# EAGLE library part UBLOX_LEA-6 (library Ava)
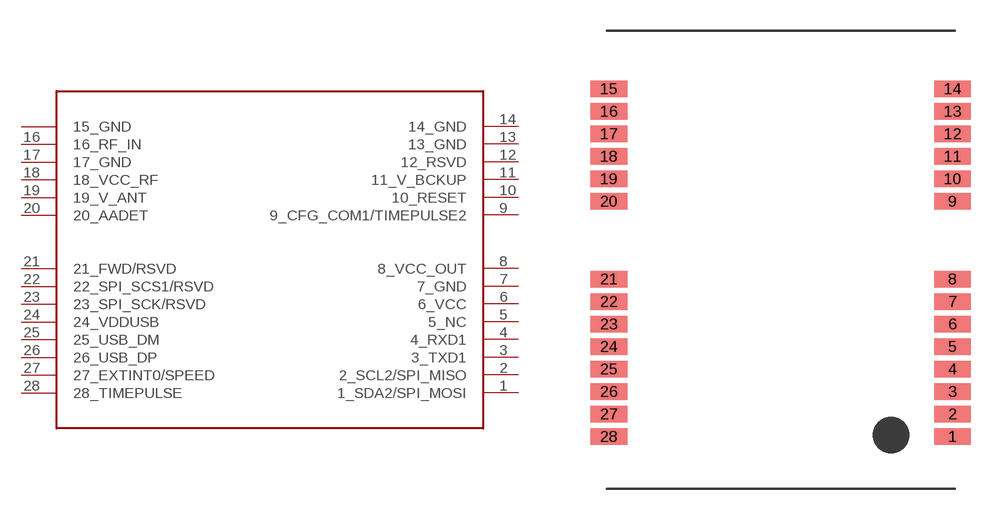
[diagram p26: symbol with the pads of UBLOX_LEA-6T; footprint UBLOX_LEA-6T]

Designator prefix -

## UBLOX_LEA-6  [UBLOX_LEA-6T]
1  1_SDA2/SPI_MOSI
2  2_SCL2/SPI_MISO
3  3_TXD1
4  4_RXD1
5  5_NC
6  6_VCC
7  7_GND
8  8_VCC_OUT
9  9_CFG_COM1/TIMEPULSE2
10  10_RESET
11  11_V_BCKUP
12  12_RSVD
13  13_GND
14  14_GND
15  15_GND
16  16_RF_IN
17  17_GND
18  18_VCC_RF
19  19_V_ANT
20  20_AADET
21  21_FWD/RSVD
22  22_SPI_SCS1/RSVD
23  23_SPI_SCK/RSVD
24  24_VDDUSB
25  25_USB_DM
26  26_USB_DP
27  27_EXTINT0/SPEED
28  28_TIMEPULSE

## Footprint UBLOX_LEA-6T (pad centres in mm)
smd 1.8 x 0.8: 1 8.4,-8.65; 2 8.4,-7.55; 3 8.4,-6.45; 4 8.4,-5.35; 5 8.4,-4.25; 6 8.4,-3.15; 7 8.4,-2.05; 8 8.4,-0.95; 9 8.4,2.85; 10 8.4,3.95; 11 8.4,5.05; 12 8.4,6.15; 13 8.4,7.25; 14 8.4,8.35; 15 -8.4,8.35; 16 -8.4,7.25; 17 -8.4,6.15; 18 -8.4,5.05; 19 -8.4,3.95; 20 -8.4,2.85; 21 -8.4,-0.95; 22 -8.4,-2.05; 23 -8.4,-3.15; 24 -8.4,-4.25; 25 -8.4,-5.35; 26 -8.4,-6.45; 27 -8.4,-7.55; 28 -8.4,-8.65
